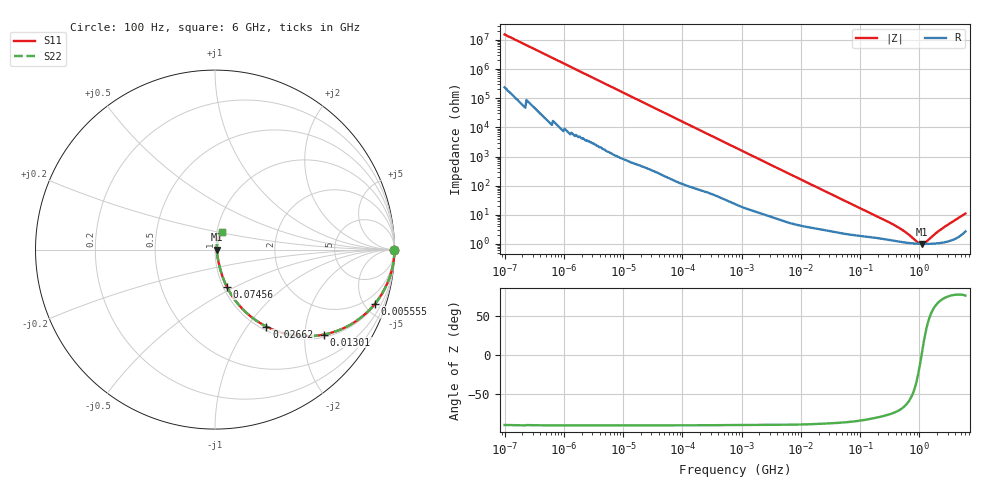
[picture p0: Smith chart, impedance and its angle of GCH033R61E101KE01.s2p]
!Murata Part Number: GCH033R61E101KE01
!These Parameters are Measured in Series Mode Connection
!Data Generated on Mar 13, 2026
!  o--ll--o
!Port1  Port2
!  o------o
!Operation Temp=25[degC], DC Bias Voltage=0[V]
!Freq. Start=100[Hz] Stop=6[GHz] 401[Steps]
# Hz S RI R 50
!Freq.(Hz) S11(Real) S11(Imag) S21(Real) S21(Imag) S12(Real) S12(Imag) S22(Real) S22(Imag)
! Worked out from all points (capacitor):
!   401 points, 100 Hz to 6 GHz, reference 50 ohm
!   read as one part in series: C = 103 pF near 109 Hz
!   lowest |Z| = 1.01 ohm at 1.095 GHz (marker M1)
!   series resonance near 1.092 GHz, so ESL is about 210 pH
!   S11 on the Smith chart (normalised r, x): 100 Hz: open; 5.555 MHz: 1.12, -5.84; 13.01 MHz: 1.08, -2.51; 26.62 MHz: 1.06, -1.24; 74.56 MHz: 1.04, -0.45; 6 GHz: 1.05, +0.21
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100  1 -6.5e-06  1e-07 6.5e-06  1e-07 6.5e-06  1 -6.5e-06
1404  1 -9.03e-05  5e-07 9.03e-05  5e-07 9.03e-05  1 -9.03e-05
1606  1 -0.000103  6e-07 0.000103  6e-07 0.000103  1 -0.000103
2008  1 -0.000129  7e-07 0.000129  7e-07 0.000129  1 -0.000129
40335  1 -0.00257  2.38e-05 0.00257  2.38e-05 0.00257  1 -0.00257
774597  0.9971 -0.0483  0.00289 0.0483  0.00289 0.0483  0.9971 -0.0483
2268635  0.9785 -0.1377  0.0215 0.1377  0.0215 0.1377  0.9785 -0.1377
5554849  0.8902 -0.3029  0.1098 0.3029  0.1098 0.3029  0.8902 -0.3029
8311524  0.7875 -0.3975  0.2125 0.3975  0.2125 0.3975  0.7875 -0.3975
1.300572e7  0.6088 -0.4731  0.3912 0.4731  0.3912 0.4731  0.6088 -0.4731
1.555665e7  0.5246 -0.4827  0.4754 0.4827  0.4754 0.4827  0.5246 -0.4827
2.662322e7  0.2869 -0.4293  0.7131 0.4293  0.7131 0.4293  0.2869 -0.4293
4.35672e7  0.1428 -0.3196  0.8572 0.3196  0.8572 0.3196  0.1428 -0.3196
7.455971e7  0.0654 -0.2062  0.9346 0.2062  0.9346 0.2062  0.0654 -0.2062
1.459435e8  0.0296 -0.1108  0.9704 0.1108  0.9704 0.1108  0.0296 -0.1108
3.124326e8  0.0162 -0.0517  0.9838 0.0517  0.9838 0.0517  0.0162 -0.0517
5.59173e8  0.0117 -0.0242  0.9883 0.0242  0.9883 0.0242  0.0117 -0.0242
9.569533e8  0.0101 -0.00455  0.9899 0.00455  0.9899 0.00455  0.0101 -0.00455
1.094528e9  0.00998 8.95e-05  0.99 -8.95e-05  0.99 -8.95e-05  0.00998 8.95e-05
1.309207e9  0.00999 0.00634  0.99 -0.00634  0.99 -0.00634  0.00999 0.00634
2.679998e9  0.0127 0.0362  0.9873 -0.0362  0.9873 -0.0362  0.0127 0.0362
6e9  0.0368 0.1008  0.9632 -0.1008  0.9632 -0.1008  0.0368 0.1008
